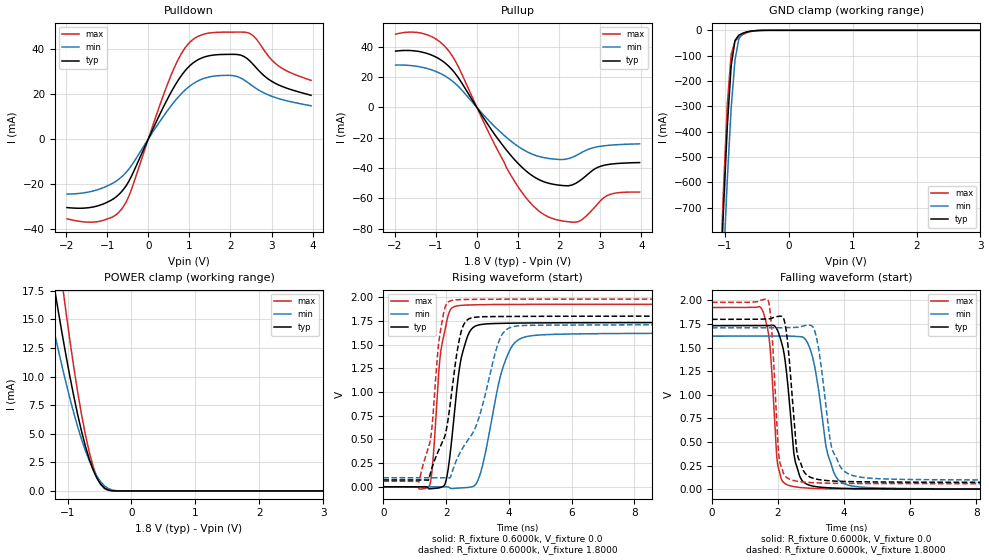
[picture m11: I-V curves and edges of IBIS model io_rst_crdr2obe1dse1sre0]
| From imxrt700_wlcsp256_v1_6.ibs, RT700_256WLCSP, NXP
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[Model] io_rst_crdr2obe1dse1sre0
|   Model io_rst_crdr2obe1dse1sre0
| This model was characterised for following simulation conditions:
| External (pad) voltage:
|   - Typ: 1.8V,   - Min: 1.71V,   - Max: 1.98V
| Library cells for typ/min/max conditions are connected as defined below:
|  PAD_RST - External Pad
|  ipp_do - Core Input
|  ipp_obe - Output Buffer Enable
|  ASRCN3V3[3] - NC
|  ASRCN3V3[4] - NC
|  ASRCP3V3[4] - NC
|  REFAPBIAS3V3 - gnde
|  REFBAMPL3V3 - vdd1v8
|  REFCAMPH3V3 - vdd1v8
|  REFDNBIAS3V3 - vdd1v8
|  REFH3V3 - REFH3V3
|  REFL3V3 - REFL3V3
|  gnde - gnde
|  ipp_dse - vdd
|  ipp_ina235_3v - NC
|  ipp_ina40_3v - NC
|  ipp_ina_mux - NC
|  ipp_ind - NC
|  ipp_ind_1p8v - NC
|  ipp_ind_3v - NC
|  ipp_sre - gnde
|  vdd - vdd
|  vdd1v8 - vdd1v8
|  vdda - vdde3v3
|  vdde3v3 - vdde3v3
| All other pins connected to ground
Model_type I/O
Polarity   Non-Inverting
Enable   Active-High
Vinl =   0.5400V
Vinh =   1.2600V
Vmeas =  0.9000V
Cref =   15.0000pF
Rref =   0.6000k
Vref =   0.0V
C_comp   3.9797pF   3.7947pF   4.1049pF
|C_comp_pullup   0.4869pF   0.5824pF   0.4755pF
|C_comp_pulldown   2.0821pF   2.1673pF   1.8518pF
[Model Spec]
| variable   typ   min   max
Vinh   1.2600V   NA   NA
Vinl   0.5400V   NA   NA
Vref   0.0V   0.0V   0.0V
Cref   15.0000pF   15.0000pF   15.0000pF
Rref   0.6000k   0.6000k   0.6000k
[Receiver Thresholds]
Vcross_high  =   0.0V
Vcross_low  =   0.0V
Vdiff_ac  =   0.0V
Vdiff_dc  =   0.0V
Tdiffslew_ac  =   0.0S
[Temperature Range]   25.0000   0.1250k   -40.0000
[Voltage Range]   1.8000V   1.7100V   1.9800V
[Pullup Reference]   1.8000V   1.7100V   1.9800V
[Pulldown Reference]   0.0V   0.0V   0.0V
[POWER Clamp Reference]   1.8000V   1.7100V   1.9800V
[GND Clamp Reference]   0.0V   0.0V   0.0V
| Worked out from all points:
|   slope of the pulldown table from 0 to 0.27 V, typ, clamps not added: 25.6 ohm
|   slope of the pullup table from 0 to 0.27 V, typ, clamps not added: 23.8 ohm
|   GND clamp passes 1 mA (typ) near -0.50 V on its own axis
|   POWER clamp passes 1 mA (typ) near -0.53 V on its own axis
|   rising waveform, R_fixture 0.6000k, V_fixture 0.0: 20-80 % time 373ps typ, 621ps min, 283ps max; typ from 0 V to 1.73 V
|   rising waveform, R_fixture 0.6000k, V_fixture 1.8000: 20-80 % time 556ps typ, 1ns min, 331ps max; typ from 0.072 V to 1.8 V
|   falling waveform, R_fixture 0.6000k, V_fixture 0.0: 20-80 % time 289ps typ, 437ps min, 205ps max; typ from 1.73 V to 0 V
|   falling waveform, R_fixture 0.6000k, V_fixture 1.8000: 20-80 % time 244ps typ, 372ps min, 176ps max; typ from 1.8 V to 0.072 V
[Pulldown]
|Voltage   I(typ)   I(min)   I(max)
-1.98V    -30.4mA    -24.44mA   -35.4mA
-1.2V     -29.49mA   -22.29mA   -36.54mA
-840mV    -26.45mA   -19.34mA   -34.25mA
-600mV    -22.26mA   -15.94mA   -29.79mA
-420mV    -16.87mA   -12.03mA   -22.87mA
600mV     22.22mA    15.79mA    30.28mA
900mV     30.36mA    21.79mA    40.52mA
1.14V     34.38mA    25.06mA    44.79mA
1.98V     37.51mA    28.2mA     47.38mA
2.46V     34.79mA    24.52mA    46.85mA
3.12V     24.4mA     18.2mA     33.06mA
3.96V     19.37mA    14.7mA     25.97mA
[Pullup]
|Voltage   I(typ)   I(min)   I(max)
-1.98V    37.17mA    27.99mA    48.3mA
-1.26V    36mA       26.04mA    48.37mA
-720mV    28.06mA    19.81mA    38.46mA
-480mV    20.65mA    14.61mA    28.37mA
780mV     -30.13mA   -21.13mA   -42.58mA
1.2V      -41.94mA   -28.92mA   -59.68mA
1.62V     -48.87mA   -33.02mA   -70.4mA
2.16V     -51.62mA   -34.11mA   -75.13mA
2.46V     -49.1mA    -31.02mA   -75.32mA
2.88V     -40.32mA   -26.22mA   -65.36mA
3.18V     -37.66mA   -25.01mA   -57.94mA
3.96V     -36.33mA   -23.97mA   -55.79mA
[GND_clamp]
|Voltage   I(typ)   I(min)   I(max)
-1.98V    -7.543A    -7.6A      -7.897A
-1.08V    -1.077A    -1.286A    -1.025A
-1.02V    -705.3mA   -921.3mA   -628.8mA
-960mV    -377.1mA   -587.4mA   -291.7mA
-900mV    -139.2mA   -307mA     -94.38mA
-840mV    -40.12mA   -117mA     -42.82mA
-780mV    -18.81mA   -33.95mA   -26.13mA
-720mV    -11.86mA   -11.44mA   -16.78mA
-660mV    -7.061mA   -5.737mA   -9.992mA
-540mV    -1.684mA   -1.901mA   -2.15mA
-420mV    -207.1uA   -403.7uA   -160.6uA
3.96V     0A         0A         0A
[POWER_clamp]
|Voltage   I(typ)   I(min)   I(max)
-1.98V    46.79mA    35.94mA    61.38mA
-1.32V    21.77mA    16.85mA    28.91mA
-1.2V     17.57mA    13.71mA    23.33mA
-1.14V    15.55mA    12.2mA     20.62mA
-1.08V    13.59mA    10.75mA    17.99mA
-1.02V    11.7mA     9.353mA    15.46mA
-900mV    8.209mA    6.76mA     10.73mA
-720mV    3.898mA    3.511mA    4.887mA
-540mV    1.103mA    1.267mA    1.195mA
-420mV    244.5uA    429.3uA    190.6uA
-180mV    280.9nA    5.273uA    26.8nA
3.96V     0A         0A         0A
[Ramp]
| variable   typ   min   max
dV/dt_r  1.0396/0.3733n   0.9730/0.6208n   1.1554/0.2834n
dV/dt_f  1.0366/0.2436n   0.9689/0.3722n   1.1528/0.1763n
R_load = 0.6000k
[Rising Waveform]
R_fixture= 0.6000k
V_fixture= 0.0
V_fixture_min= 0.0
V_fixture_max= 0.0
|time   V(typ)   V(min)   V(max)
0s        47.1nV     1.315uV    17.96nV
1.472ns   -22.05mV   -567.9uV   13.97mV
1.568ns   -18.72mV   -624.2uV   227.8mV
1.861ns   -2.625mV   -472.5uV   1.494V
2.072ns   200.9mV    -2.395mV   1.815V
2.442ns   1.286V     -13.7mV    1.913V
3.053ns   1.708V     100.6mV    1.92V
3.999ns   1.725V     1.419V     1.923V
4.898ns   1.729V     1.599V     1.924V
60ns      1.733V     1.622V     1.926V
[Rising Waveform]
R_fixture= 0.6000k
V_fixture= 1.8000
V_fixture_min= 1.7100
V_fixture_max= 1.9800
|time   V(typ)   V(min)   V(max)
0s        72.29mV    95.11mV    58.66mV
1.137ns   71.88mV    95.04mV    54.48mV
1.518ns   167.5mV    94.57mV    533.8mV
1.75ns    374.5mV    94.76mV    1.477V
1.907ns   489.9mV    94.93mV    1.813V
2.324ns   1.371V     275.6mV    1.972V
2.705ns   1.767V     496.9mV    1.976V
3.703ns   1.796V     1.553V     1.979V
4.344ns   1.797V     1.698V     1.979V
60ns      1.8V       1.71V      1.98V
[Falling Waveform]
R_fixture= 0.6000k
V_fixture= 0.0
V_fixture_min= 0.0
V_fixture_max= 0.0
|time   V(typ)   V(min)   V(max)
0s        1.733V     1.622V     1.926V
1.533ns   1.734V     1.622V     1.892V
1.748ns   1.733V     1.621V     1.546V
1.962ns   1.699V     1.622V     350.2mV
2.191ns   1.419V     1.623V     64.36mV
2.694ns   110.2mV    1.616V     16.72mV
3.051ns   32.74mV    1.392V     8.782mV
3.685ns   11.82mV    183.1mV    3.436mV
4.536ns   5.176mV    21.44mV    1.187mV
60ns      2.732uV    5.895uV    307nV
[Falling Waveform]
R_fixture= 0.6000k
V_fixture= 1.8000
V_fixture_min= 1.7100
V_fixture_max= 1.9800
|time   V(typ)   V(min)   V(max)
0s        1.8V       1.71V      1.98V
1.708ns   1.804V     1.71V      1.994V
2.023ns   1.833V     1.71V      359.6mV
2.159ns   1.817V     1.711V     174mV
2.57ns    401.4mV    1.715V     84.63mV
2.799ns   178.5mV    1.733V     74.32mV
3.168ns   105.7mV    1.603V     66.68mV
3.662ns   86.64mV    400.2mV    62.41mV
4.773ns   76.82mV    116.6mV    59.61mV
60ns      72.29mV    95.11mV    58.66mV
